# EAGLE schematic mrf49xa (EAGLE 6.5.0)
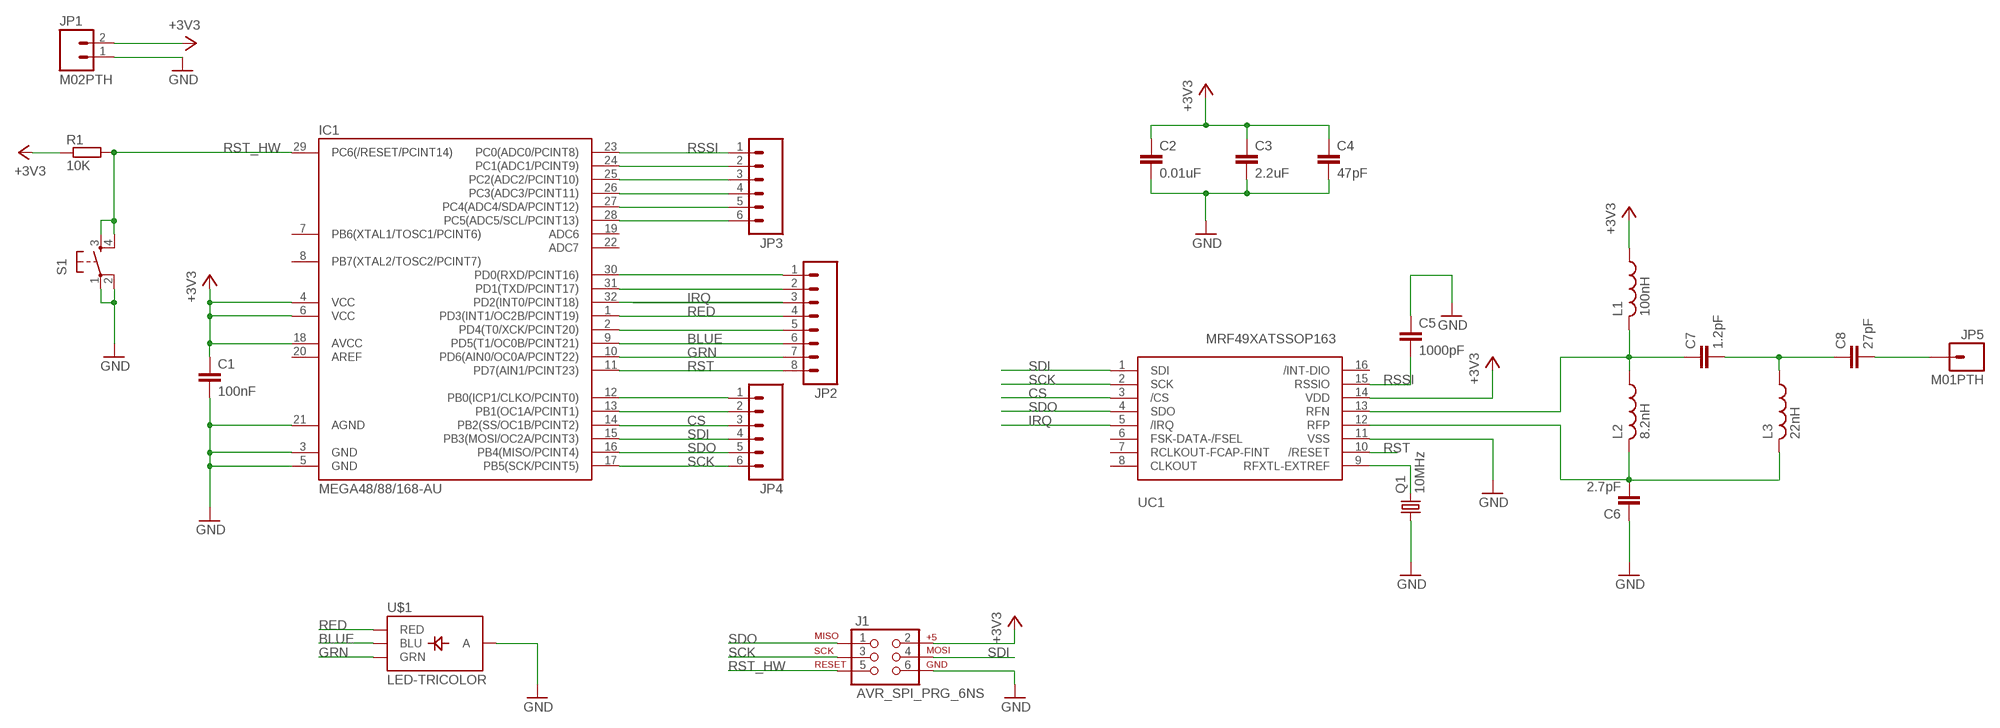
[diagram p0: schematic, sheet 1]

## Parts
C1  100nF  C-EUC0805  [C0805]
C2  0.01uF  C-EUC0603  [C0603]
C3  2.2uF  C-EUC1206  [C1206]
C4  47pF  C-EUC0603  [C0603]
C5  1000pF  C-EUC1206  [C1206]
C6  2.7pF  C-EUC1206  [C1206]
C7  1.2pF  C-EUC1206  [C1206]
C8  27pF  C-EUC1206  [C1206]
IC1  MEGA48/88/168-AU  [TQFP32-08]
J1  AVR_SPI_PRG_6NS  [2X3-NS]
JP1  M02PTH  [1X02]
JP2  M08  [1X08_PIN1_NO_SILK]
JP3  M06SIP  [1X06]
JP4  M06SIP  [1X06]
JP5  M01PTH  [1X01]
L1  100nH  L-USL3216C  [L3216C]
L2  8.2nH  L-USL3225P  [L3225P]
L3  22nH  L-USL3225P  [L3225P]
Q1  10MHz  CRYSTALSMD  [HC49UP]
R1  10K  R-EU_R2012  [R2012]
S1  TAC_SWITCHSMD  [TACTILE_SWITCH_SMD]
U$1  LED-TRICOLOR  [LED-TRICOLOR-SMD]
UC1  MRF49XATSSOP163  [TSSOP16]

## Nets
+3V3: C1.1 C2.1 C3.1 C4.1 IC1.4(VCC) IC1.6(VCC) IC1.18(AVCC) J1.2 JP1.2 L1.1 R1.1 UC1.14(VDD)
BLUE: IC1.9(PD5(T1/OC0B/PCINT21)) JP2.6 U$1.B(BLU)
CS: IC1.14(PB2(SS/OC1B/PCINT2)) JP4.3 UC1.3(/CS)
GND: C1.2 C2.2 C3.2 C4.2 C5.1 C6.1 IC1.3(GND) IC1.5(GND) IC1.21(AGND) J1.6 JP1.1 Q1.1 S1.1 S1.2 U$1.A UC1.11(VSS)
GRN: IC1.10(PD6(AIN0/OC0A/PCINT22)) JP2.7 U$1.G(GRN)
IRQ: IC1.32(PD2(INT0/PCINT18)) JP2.3 UC1.5(/IRQ)
N$1: IC1.24(PC1(ADC1/PCINT9)) JP3.2
N$2: IC1.25(PC2(ADC2/PCINT10)) JP3.3
N$3: IC1.26(PC3(ADC3/PCINT11)) JP3.4
N$4: IC1.27(PC4(ADC4/SDA/PCINT12)) JP3.5
N$5: IC1.28(PC5(ADC5/SCL/PCINT13)) JP3.6
N$6: IC1.30(PD0(RXD/PCINT16)) JP2.1
N$8: IC1.31(PD1(TXD/PCINT17)) JP2.2
N$9: Q1.2 UC1.9(RFXTL-EXTREF)
N$10: C7.1 L1.2 L2.1 UC1.13(RFN)
N$11: C7.2 C8.1 L3.1
N$12: C6.2 L2.2 L3.2 UC1.12(RFP)
N$13: C8.2 JP5.1
N$16: IC1.2(PD4(T0/XCK/PCINT20)) JP2.5
N$20: IC1.12(PB0(ICP1/CLKO/PCINT0)) JP4.1
N$21: IC1.13(PB1(OC1A/PCINT1)) JP4.2
RED: IC1.1(PD3(INT1/OC2B/PCINT19)) JP2.4 U$1.R(RED)
RSSI: C5.2 IC1.23(PC0(ADC0/PCINT8)) JP3.1 UC1.15(RSSIO)
RST: IC1.11(PD7(AIN1/PCINT23)) JP2.8 UC1.10(/RESET)
RST_HW: IC1.29(PC6(/RESET/PCINT14)) J1.5 R1.2 S1.3 S1.4
SCK: IC1.17(PB5(SCK/PCINT5)) J1.3 JP4.6 UC1.2(SCK)
SDI: IC1.15(PB3(MOSI/OC2A/PCINT3)) J1.4 JP4.4 UC1.1(SDI)
SDO: IC1.16(PB4(MISO/PCINT4)) J1.1 JP4.5 UC1.4(SDO)
Unconnected: IC1.7(PB6(XTAL1/TOSC1/PCINT6)) IC1.8(PB7(XTAL2/TOSC2/PCINT7)) IC1.19(ADC6) IC1.20(AREF) IC1.22(ADC7) UC1.6(FSK-DATA-/FSEL) UC1.7(RCLKOUT-FCAP-FINT) UC1.8(CLKOUT) UC1.16(/INT-DIO)

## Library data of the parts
C1-C8 = rcl:C-EU: CAPACITOR, European symbol
IC1 = avr-6:MEGA48/88/168
J1 = SparkFun-Connectors:AVR_SPI_PRG_6: AVR ISP 6 Pin This is the reduced ISP connector for AVR programming. Common on Arduino. This footprint will take up less PCB space and can be used with a 10-pin to 6-pin adapter such as SKU: BOB-08508
JP1 = SparkFun-Connectors:M02: Standard 2-pin 0.1" header. Use with
JP2 = SparkFun-Connectors:M08: Header 8 Standard 8-pin 0.1" header. Use with straight break away headers (SKU : PRT-00116), right angle break away headers (PRT-00553), swiss pins (PRT-00743), machine pins (PRT-00117), and female headers (PRT-00115).
JP3 JP4 = SparkFun-Connectors:M06: Header 6 Standard 6-pin 0.1" header. Use with straight break away headers (SKU : PRT-00116), right angle break away headers (PRT-00553), swiss pins (PRT-00743), machine pins (PRT-00117), and female headers (PRT-00115). Molex polarized connector foot print use with SKU : PRT-08094 with associated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
JP5 = SparkFun-Connectors:M01: Header 1
L1-L3 = rcl:L-US: INDUCTOR, American symbol
Q1 = SparkFun:CRYSTAL: Crystals
R1 = resistor:R-EU_: RESISTOR, European symbol
S1 = SparkFun-Electromechanical:TAC_SWITCH: Momentary Switch Button commonly used for reset or general input. Spark Fun Electronics SKU : COM-00097 SMT- SWCH-08247; PROD_ID: SWCH-08247
U$1 = SparkFun-LED:LED-TRICOLOR: Tri-Color LED SMD Proven layout and schematic for triple color LED in SMD package - common anode. Spark Fun Electronics SKU : COM-07844
UC1 = nicolas:MRF49XA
